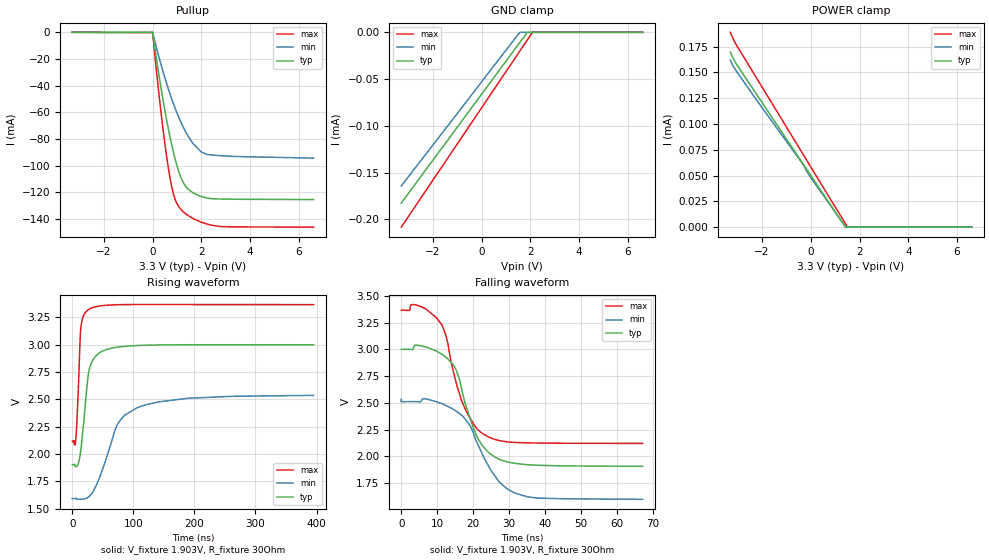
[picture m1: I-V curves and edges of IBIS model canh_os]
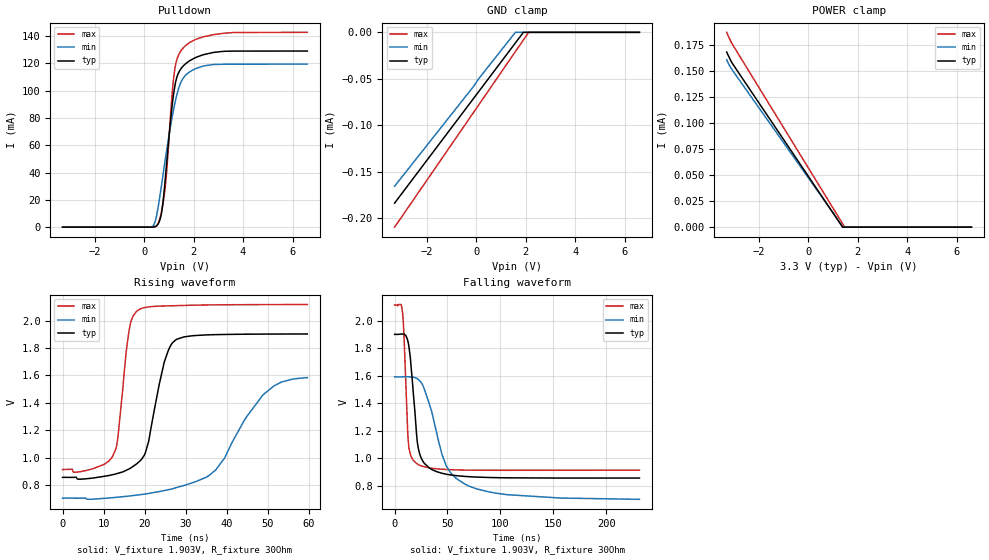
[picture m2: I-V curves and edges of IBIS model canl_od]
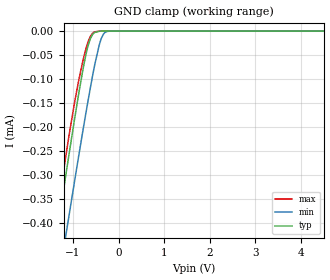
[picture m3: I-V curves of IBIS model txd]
|Texas Instruments Incorporated
| TCAN33x 3.3-V CAN Transceivers with CAN FD (Flexible Data Rate)
| Marketing part#   Digital Voltage Range   Package-type   #pins
| TCAN330DCNR   3V-3.6V   SOT-23   8
| TCAN330DCNT   3V-3.6V   SOT-23   8
| TCAN330GDCNR   3V-3.6V   SOT-23   8
| TCAN330GDCNT   3V-3.6V   SOT-23   8
| TCAN332DCNR   3V-3.6V   SOT-23   8
| TCAN332DCNT   3V-3.6V   SOT-23   8
| TCAN332GDCNR   3V-3.6V   SOT-23   8
| TCAN332GDCNT   3V-3.6V   SOT-23   8
| TCAN334DCNR   3V-3.6V   SOT-23   8
| TCAN334DCNT   3V-3.6V   SOT-23   8
| TCAN334GDCNR   3V-3.6V   SOT-23   8
| TCAN334GDCNT   3V-3.6V   SOT-23   8
| TCAN337DCNR   3V-3.6V   SOT-23   8
| TCAN337DCNT   3V-3.6V   SOT-23   8
| TCAN337GDCNR   3V-3.6V   SOT-23   8
| TCAN337GDCNT   3V-3.6V   SOT-23   8
[IBIS Ver]   4.1
[File name]   tcan33x.ibs
[File Rev]   1.0
[Date]   06/09/2016
[Source]
| Texas Instruments Incorporated.
| Analog-eLab Design Center, HPA
| 12500 TI Blvd
| Dallas, TX -75243
[Notes]   Revision History:
| Rev 1.0: 06/09/2016
| - Initial version of the model
| - Model generated from simulations in SPECTRE
| - Model matched to SPICE simulation
| - C_comp although listed in numerical order of value are
|   obtained from varying PVT conditions. For PVT conditions for
|   each specific value refer the buffer description under
|   respective [Model]. IBIS model user is responsible for using
|   appropriate C_comp to simulate for Signal Integrity.
|* EXCEPTION:   *
|* - For s model there is leakage in power clamp due to resistor connected*
|*   to pad.   *
|* - For canh_os model pullup table does not pass through zero due to   *
|*   resistor network connected to PAD. Power clamp and ground clamp   *
|*   tables have leakage due to resistor network connected to PAD.   *
|* - For canl_od model power clamp and ground clamp table have leakage due*
|*   to resistor network connected to PAD.   *
[Disclaimer]
| This model is designed as an aid for customers of Texas Instruments.
| TI and its licensors and suppliers make no warranties, either expressed
| or implied, with respect to this  model, including the warranties of
| merchantability or fitness for a particular purpose. The model is
| provided solely on an "as is" basis. The entire risk as to its quality
| and performance is with the customer.
[Copyright]
(C) Copyright 2016 Texas Instruments Incorporated.All rights reserved.
|   TCAN330DCN
[Component]   TCAN330DCN
[Manufacturer]   TI
[Package]   |SOT-23 - DCN Package
|   typ   min   max
R_pkg   0.00644   0.00487   0.00958
L_pkg   1.07993nH   0.78642nH   1.66696nH
C_pkg   0.27013pF   0.20487pF   0.40066pF
[Pin]  signal_name   model_name   R_pin   L_pin   C_pin
1   TXD   txd   0.00487   0.78642nH  0.20487pF
2   GND   gnd   0.00958   1.66695nH  0.40066pF
3   VCC   power   0.00958   1.66696nH  0.40066pF
4   RXD   rxd   0.00487   0.78642nH  0.20487pF
5   SHDN   s   0.00487   0.78642nH  0.20487pF
6   CANL   canl_od   0.00958   1.66696nH  0.40066pF
7   CANH   canh_os   0.00958   1.66696nH  0.40066pF
8   S   s   0.00487   0.78642nH  0.20487pF
9   thermal_pad1   nc   0.00040   0.07257nH  0.05601pF
10   thermal_pad2   nc   0.00040   0.07257nH  0.05601pF
11   thermal_pad3   nc   0.00040   0.07257nH  0.05601pF
12   thermal_pad4   nc   0.00040   0.07257nH  0.05601pF
[Diff_pin]   inv_pin   vdiff   tdelay_typ   tdelay_min   tdelay_max
7   6   NA   NA   NA   NA
|   TCAN332DCN
[Component]   TCAN332DCN
[Manufacturer]   TI
[Package]   |SOT-23 - DCN Package
|   typ   min   max
R_pkg   0.007225   0.00487   0.00958
L_pkg   1.22669nH   0.78642nH   1.66696nH
C_pkg   0.302765pF   0.20487pF   0.40066pF
[Pin]  signal_name   model_name   R_pin   L_pin   C_pin
1   TXD   txd   0.00487   0.78642nH  0.20487pF
2   GND   gnd   0.00958   1.66695nH  0.40066pF
3   VCC   power   0.00958   1.66696nH  0.40066pF
4   RXD   rxd   0.00487   0.78642nH  0.20487pF
5   NC   nc   0.00487   0.78642nH  0.20487pF
6   CANL   canl_od   0.00958   1.66696nH  0.40066pF
7   CANH   canh_os   0.00958   1.66696nH  0.40066pF
8   NC   nc   0.00487   0.78642nH  0.20487pF
9   thermal_pad1   nc   0.00040   0.07257nH  0.05601pF
10   thermal_pad2   nc   0.00040   0.07257nH  0.05601pF
11   thermal_pad3   nc   0.00040   0.07257nH  0.05601pF
12   thermal_pad4   nc   0.00040   0.07257nH  0.05601pF
[Diff_pin]   inv_pin   vdiff   tdelay_typ   tdelay_min   tdelay_max
7   6   NA   NA   NA   NA
|   TCAN334DCN
[Component]   TCAN334DCN
[Manufacturer]   TI
[Package]   |SOT-23 - DCN Package
|   typ   min   max
R_pkg   0.00644   0.00487   0.00958
L_pkg   1.07993nH   0.78642nH   1.66696nH
C_pkg   0.27013pF   0.20487pF   0.40066pF
[Pin]  signal_name   model_name   R_pin   L_pin   C_pin
1   TXD   txd   0.00487   0.78642nH  0.20487pF
2   GND   gnd   0.00958   1.66695nH  0.40066pF
3   VCC   power   0.00958   1.66696nH  0.40066pF
4   RXD   rxd   0.00487   0.78642nH  0.20487pF
5   SHDN   s   0.00487   0.78642nH  0.20487pF
6   CANL   canl_od   0.00958   1.66696nH  0.40066pF
7   CANH   canh_os   0.00958   1.66696nH  0.40066pF
8   STB   s   0.00487   0.78642nH  0.20487pF
9   thermal_pad1   nc   0.00040   0.07257nH  0.05601pF
10   thermal_pad2   nc   0.00040   0.07257nH  0.05601pF
11   thermal_pad3   nc   0.00040   0.07257nH  0.05601pF
12   thermal_pad4   nc   0.00040   0.07257nH  0.05601pF
[Diff_pin]   inv_pin   vdiff   tdelay_typ   tdelay_min   tdelay_max
7   6   NA   NA   NA   NA
|   TCAN337DCN
[Component]   TCAN337DCN
[Manufacturer]   TI
[Package]   |SOT-23 - DCN Package
|   typ   min   max
R_pkg   0.00644   0.00487   0.00958
L_pkg   1.07993nH   0.78642nH   1.66696nH
C_pkg   0.27013pF   0.20487pF   0.40066pF
[Pin]  signal_name   model_name   R_pin   L_pin   C_pin
1   TXD   txd   0.00487   0.78642nH  0.20487pF
2   GND   gnd   0.00958   1.66695nH  0.40066pF
3   VCC   power   0.00958   1.66696nH  0.40066pF
4   RXD   rxd   0.00487   0.78642nH  0.20487pF
5   FAULT   fault   0.00487   0.78642nH  0.20487pF
6   CANL   canl_od   0.00958   1.66696nH  0.40066pF
7   CANH   canh_os   0.00958   1.66696nH  0.40066pF
8   S   s   0.00487   0.78642nH  0.20487pF
9   thermal_pad1   nc   0.00040   0.07257nH  0.05601pF
10   thermal_pad2   nc   0.00040   0.07257nH  0.05601pF
11   thermal_pad3   nc   0.00040   0.07257nH  0.05601pF
12   thermal_pad4   nc   0.00040   0.07257nH  0.05601pF
[Diff_pin]   inv_pin   vdiff   tdelay_typ   tdelay_min   tdelay_max
7   6   NA   NA   NA   NA
| Models and submodels in the file (6): canh_os (Open_source), canl_od (Open_drain), txd (Input), s (Input), rxd (Output), fault (Open_drain)
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|   canh_os Model
[Model]   canh_os
Model_type   Open_source
Polarity   Inverting
Vmeas = 2.448
Vref = 1.903
Cref = 2pF
Rref = 30
|   typ   min   max
|   (nom PVT)   (fast PVT)   (slow PVT)
C_comp   8.774e-12   8.279e-12   9.313e-12
| Where nom  PVT is Nominal Process, 3.3V, 27C
|   Fast PVT is Strong Process,  3.6V, -40C
|   Slow PVT is Weak Process,   3V, 150C
[Voltage Range]   3.3   3   3.6
|Junction Temperature
[Temperature Range]   27   150   -40
[Pullup Reference]   3.3   3   3.6
[Pulldown Reference]   0   0   0
[Power Clamp Reference]   3.3   3   3.6
[GND Clamp Reference]   0   0   0
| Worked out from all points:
|   slope of the pullup table from 0 to 0.495 V, typ, clamps not added: 8.61 ohm
|   falling waveform, V_fixture 1.903V, R_fixture 30Ohm: 20-80 % time 6.54ns typ, 8.9ns min, 6.37ns max; typ from 3 V to 1.91 V
|   rising waveform, V_fixture 1.903V, R_fixture 30Ohm: 20-80 % time 12.3ns typ, 40.2ns min, 5.32ns max; typ from 1.9 V to 3 V
[GND Clamp]
|   Voltage   I(typ)   I(min)   I(max)
-3.3V     -182.6uA   -164.3uA   -208.4uA
1.56V     -10.9uA    -90.42nA   -20.16uA
1.868V    -18.09nA   0A         -8.24uA
2.082V    0A         0A         0A
6.6V      0A         0A         0A
[Pullup]
|   Voltage   I(typ)   I(min)   I(max)
-3.3V     48.55nA    67.8nA     46.35nA
-2.4mV    -115.6uA   -44.14uA   -224.6uA
387mV     -46.57mA   -27.01mA   -67mA
564.3mV   -64.89mA   -37.89mA   -92.05mA
703.2mV   -77.79mA   -45.78mA   -108.3mA
825mV     -87.93mA   -52.2mA    -119.2mA
960.3mV   -97.74mA   -58.8mA    -127mA
1.155V    -108.7mA   -67.26mA   -132.6mA
1.359V    -115.7mA   -74.81mA   -136.1mA
1.67V     -120.5mA   -83.69mA   -139.7mA
2.204V    -124.1mA   -91.34mA   -143.6mA
6.6V      -125.4mA   -94.3mA    -146.1mA
[POWER Clamp]
|   Voltage   I(typ)   I(min)   I(max)
-3.3V     169.7uA    161.8uA    188.7uA
-3.175V   163.3uA    155.8uA    182uA
-3.036V   157.5uA    150.7uA    176uA
-2.169V   126.8uA    121.4uA    142.4uA
-291mV    60.45uA    60.05uA    69.65uA
-168mV    56.13uA    54.34uA    64.88uA
-3mV      50.27uA    48.21uA    58.49uA
739.2mV   24.04uA    23.33uA    29.74uA
1.426V    0A         192.7nA    3.36uA
1.513V    0A         0A         0A
6.6V      0A         0A         0A
[Ramp]
R_load = 30
|   typ   min   max
dV/dt_r   0.6581/1.23427e-08   0.566485/4.00658e-08   0.75016/5.27908e-09
dV/dt_f   0.658458/6.55213e-09   0.550194/8.57309e-09   0.750563/6.41211e-09
[Falling Waveform]
V_fixture = 1.903V
V_fixture_min = 1.593V
V_fixture_max = 2.117V
R_fixture = 30Ohm
|   Time   V(typ)   V(min)   V(max)
0s        3V         2.533V     3.368V
4.014ns   3.04V      2.512V     3.417V
9.955ns   2.982V     2.509V     3.29V
12.49ns   2.925V     2.474V     3.124V
14.45ns   2.857V     2.439V     2.799V
17.64ns   2.513V     2.354V     2.454V
23.31ns   2.07V      1.968V     2.198V
27.62ns   1.966V     1.747V     2.144V
34.8ns    1.921V     1.623V     2.125V
67.2ns    1.906V     1.597V     2.12V
[Rising Waveform]
V_fixture = 1.903V
V_fixture_min = 1.593V
V_fixture_max = 2.117V
R_fixture = 30Ohm
|   Time   V(typ)   V(min)   V(max)
0s        1.903V     1.593V     2.117V
6.218ns   1.886V     1.593V     2.159V
13.13ns   1.997V     1.587V     3.075V
14.49ns   2.052V     1.588V     3.173V
24.78ns   2.659V     1.601V     3.313V
28.88ns   2.796V     1.62V      3.33V
44.07ns   2.925V     1.775V     3.354V
72.89ns   2.978V     2.26V      3.366V
105.4ns   2.993V     2.422V     3.368V
395.2ns   3V         2.537V     3.367V
|   canl_od Model
[Model]   canl_od
Model_type   Open_drain
Polarity   Non-Inverting
Vmeas = 1.372
Vref = 1.903
Cref = 2pF
Rref = 30
|   typ   min   max
|   (nom PVT)   (fast PVT)   (slow PVT)
C_comp   7.409e-12   2.536e-17   1.206e-11
| Where nom  PVT is Nominal Process, 3.3V, 27C
|   Fast PVT is Strong Process,  3.6V, -40C
|   Slow PVT is Weak Process,   3V, 150C
[Voltage Range]   3.3   3   3.6
|Junction Temperature
[Temperature Range]   27   150   -40
[Pullup Reference]   3.3   3   3.6
[Pulldown Reference]   0   0   0
[Power Clamp Reference]   3.3   3   3.6
[GND Clamp Reference]   0   0   0
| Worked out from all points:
|   slope of the pulldown table from 0 to 0.495 V, typ, clamps not added: 556 ohm
|   falling waveform, V_fixture 1.903V, R_fixture 30Ohm: 20-80 % time 7.29ns typ, 22.8ns min, 3.71ns max; typ from 1.9 V to 0.855 V
|   rising waveform, V_fixture 1.903V, R_fixture 30Ohm: 20-80 % time 4.28ns typ, 11.5ns min, 2.46ns max; typ from 0.855 V to 1.9 V
[Pulldown]
|   Voltage   I(typ)   I(min)   I(max)
-3.3V     -481.2nA   -44.25nA   -71.61nA
300mV     19.96uA    233uA      7.353uA
441mV     345.7uA    3.704mA    240.2uA
562.8mV   2.267mA    14.22mA    2.388mA
722.7mV   12.62mA    33.19mA    13.22mA
858mV     36.03mA    49.91mA    29.94mA
1.104V    84.37mA    77.72mA    91.22mA
1.24V     103.1mA    90.42mA    115.7mA
1.396V    113.2mA    101.6mA    126.2mA
1.693V    120mA      111.7mA    133.3mA
3.227V    128.8mA    119.3mA    142.1mA
6.6V      129mA      119.5mA    142.7mA
[GND Clamp]
|   Voltage   I(typ)   I(min)   I(max)
-3.3V     -184uA     -165.9uA   -210uA
-180mV    -73.8uA    -60.69uA   -89.13uA
138mV     -62.55uA   -48.78uA   -76.81uA
1.584V    -11.44uA   0A         -20.77uA
1.907V    -8.816nA   0A         -8.239uA
2.122V    0A         0A         0A
6.6V      0A         0A         0A
[POWER Clamp]
|   Voltage   I(typ)   I(min)   I(max)
-3.3V     168.5uA    161uA      187.4uA
-3.175V   162.1uA    155uA      180.7uA
-3.034V   156.2uA    149.8uA    174.5uA
1.383V    107.8nA    920.6nA    3.487uA
1.41V     0A         0A         2.43uA
1.474V    0A         0A         0A
6.6V      0A         0A         0A
[Ramp]
R_load = 30
|   typ   min   max
dV/dt_r   0.628725/4.23394e-09   0.533683/1.14069e-08   0.722799/2.44452e-09
dV/dt_f   0.628353/7.28685e-09   0.536847/2.27906e-08   0.722213/3.70322e-09
[Falling Waveform]
V_fixture = 1.903V
V_fixture_min = 1.593V
V_fixture_max = 2.117V
R_fixture = 30Ohm
|   Time   V(typ)   V(min)   V(max)
0s        1.903V     1.593V     2.117V
7.536ns   1.905V     1.594V     2.06V
8.689ns   1.905V     1.594V     1.922V
12.74ns   1.847V     1.594V     1.143V
15.59ns   1.665V     1.593V     1.014V
21.5ns    1.115V     1.579V     958.3mV
28.49ns   959.4mV    1.496V     936.8mV
48.83ns   883.2mV    944.2mV    917.8mV
65.88ns   867.5mV    813.9mV    913.5mV
231.4ns   855.2mV    700.1mV    912.5mV
[Rising Waveform]
V_fixture = 1.903V
V_fixture_min = 1.593V
V_fixture_max = 2.117V
R_fixture = 30Ohm
|   Time   V(typ)   V(min)   V(max)
0s        855.1mV    703.4mV    912.3mV
12.24ns   874.9mV    706.8mV    1.011V
13.48ns   884.6mV    710.2mV    1.144V
16.17ns   916mV      718.5mV    1.921V
18.17ns   956.4mV    725.7mV    2.072V
20.19ns   1.035V     733.7mV    2.098V
27.62ns   1.861V     779.5mV    2.11V
37.35ns   1.899V     910mV      2.116V
48.98ns   1.903V     1.462V     2.118V
59.65ns   1.903V     1.584V     2.119V
|   txd Model
[Model]   txd
Model_type   Input
Vinl = 0.66
Vinh = 2.64
|   typ   min   max
|   (nom PVT)   (fast PVT)   (slow PVT)
C_comp   3.454e-13   3.262e-13   3.623e-13
[Model spec]
|subparameter
Vinl   0.66   0.60   0.72
Vinh   2.64   2.40   2.88
| Where nom  PVT is Nominal Process, 3.3V, 27C
|   Fast PVT is Strong Process,  3.6V, -40C
|   Slow PVT is Weak Process,   3V, 150C
[Voltage Range]   3.3   3   3.6
|Junction Temperature
[Temperature Range]   27   150   -40
[Power Clamp Reference]   3.3   3   3.6
[GND Clamp Reference]   0   0   0
[GND Clamp]
|   Voltage   I(typ)   I(min)   I(max)
-3.3V     -1.686mA   -1.741mA   -1.779mA
-1.626V   -597.6uA   -709.8uA   -578.6uA
-1.334V   -412uA     -533.2uA   -377.5uA
-1.165V   -305.8uA   -431.7uA   -266.4uA
-1.086V   -257.1uA   -384.8uA   -217.8uA
-877.8mV  -133.3uA   -262.8uA   -105.2uA
-726mV    -53.98uA   -176.7uA   -40.49uA
-620.4mV  -16.38uA   -119.5uA   -11.35uA
-521.4mV  -2.845uA   -69.79uA   -1.539uA
-375mV    -93.35nA   -14.46uA   -22.06nA
-217.8mV  0A         -390.2nA   0A
6.6V      0A         0A         0A
[POWER Clamp]
|   Voltage   I(typ)   I(min)   I(max)
-3.3V     0A         0A         0A
0V        0A         0A         0A
6.6V      0A         0A         0A
